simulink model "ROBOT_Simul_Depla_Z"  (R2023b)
settings: Solver=ode15s  StartTime=0.0  StopTime=0.2  RelTol=1e-3  EnableMultiTasking=on
undefined symbols (not defined in the file): BATI1_Défaut_sldprt, BATI2_Défaut_sldprt, BATI3_Défaut_sldprt, deg, kg, m, mm, N, rad, s, STL, X, Y, Z
libraries: sm_lib x139, fl_lib x42, nesl_utility x19, slpidlib x3
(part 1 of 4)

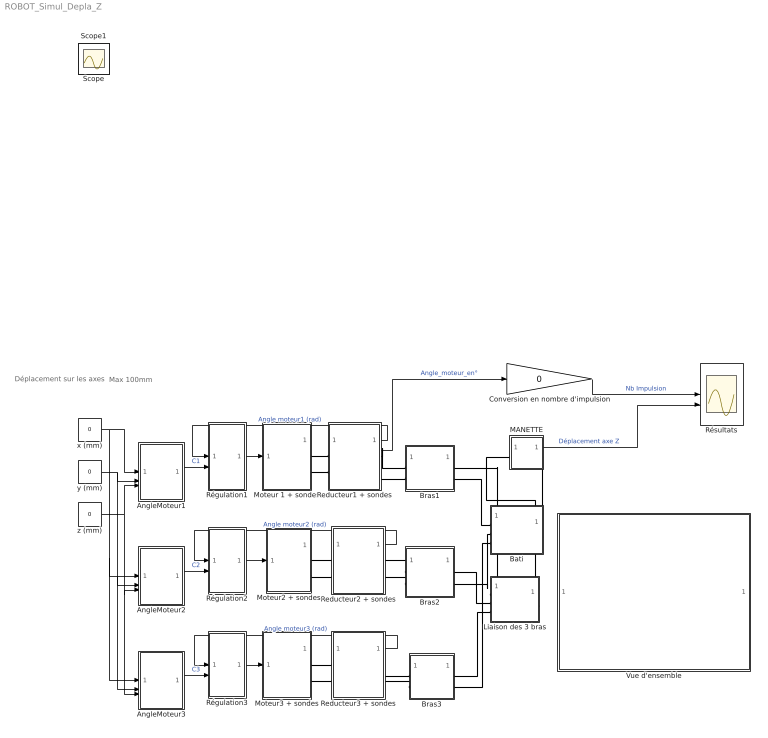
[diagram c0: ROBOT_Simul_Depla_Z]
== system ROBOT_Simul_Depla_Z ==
  note: Déplacement sur les axes
  note: Max 100mm
  AngleMoteur1 : MATLAB Function  TreatAsAtomicUnit=on
  AngleMoteur2 : MATLAB Function  TreatAsAtomicUnit=on
  AngleMoteur3 : MATLAB Function  TreatAsAtomicUnit=on
  Bati : Subsystem
  Bras1 : Subsystem
  Bras2 : Subsystem
  Bras3 : Subsystem
  Conversion en nombre d'impulsion : Gain  Gain=0
  Liaison des 3 bras : Subsystem
  MANETTE : Subsystem
  Moteur 1 + sondes : Subsystem
  Moteur2 + sondes : Subsystem
  Moteur3 + sondes : Subsystem
  Reducteur1 + sondes : Subsystem
  Reducteur2 + sondes : Subsystem
  Reducteur3 + sondes : Subsystem
  Régulation1 : Subsystem
  Régulation2 : Subsystem
  Régulation3 : Subsystem
  Résultats : Scope  NumInputPorts=2
  Vue d'ensemble : Subsystem
  x (mm) : Constant  Value=0
  y (mm) : Constant  Value=0
  z (mm) : Constant  Value=0
  Scope : Scope
  Scope1 : Scope
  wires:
  Régulation3/1(Out1) -> Moteur3 + sondes/1(In1)
  Reducteur3 + sondes/1(Angle_mot3) -> Régulation3/1(In1)  "Angle moteur3 (rad)"
  Régulation1/1(Out1) -> Moteur 1 + sondes/1(In1)
  Reducteur1 + sondes/1(Angle_mot1) -> Régulation1/1(In1)  "Angle moteur1 (rad)"
  Régulation2/1(Out1) -> Moteur2 + sondes/1(In1)
  Reducteur2 + sondes/1(Angle_mot2) -> Régulation2/1(In1)  "Angle moteur2 (rad)"
  AngleMoteur3/1(anglmot3) -> Régulation3/2(In2)  "C3"
  x (mm)/1 -> AngleMoteur1/1(x), AngleMoteur2/1(x), AngleMoteur3/1(x)
  AngleMoteur1/1(anglmot1) -> Régulation1/2(In2)  "C1"
  AngleMoteur2/1(anglmot2) -> Régulation2/2(In2)  "C2"
  y (mm)/1 -> AngleMoteur1/2(y), AngleMoteur2/2(y), AngleMoteur3/2(y)
  z (mm)/1 -> AngleMoteur1/3(z), AngleMoteur2/3(z), AngleMoteur3/3(z)
  Reducteur1 + sondes/2(Angle_mot_°) -> Conversion en nombre d'impulsion/1  "Angle_moteur_en°"
  Conversion en nombre d'impulsion/1 -> Résultats/1  "Nb Impulsion"
  MANETTE/1(Out1) -> Résultats/2  "Déplacement axe Z"
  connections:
  Liaison des 3 bras/RConn1 -- MANETTE/LConn1
  Moteur3 + sondes/RConn1 -- Reducteur3 + sondes/LConn1
  Moteur 1 + sondes/RConn1 -- Reducteur1 + sondes/LConn1
  Moteur3 + sondes/RConn2 -- Reducteur3 + sondes/LConn2
  Reducteur1 + sondes/LConn2 -- Moteur 1 + sondes/RConn2
  Moteur2 + sondes/RConn2 -- Reducteur2 + sondes/LConn2
  Moteur2 + sondes/RConn1 -- Reducteur2 + sondes/LConn1
  Reducteur1 + sondes/RConn1 -- Bras1/LConn1
  Reducteur1 + sondes/RConn2 -- Bras1/LConn2
  Liaison des 3 bras/LConn1 -- Bras1/RConn1
  Liaison des 3 bras/LConn2 -- Bras2/RConn1
  Bras2/LConn1 -- Reducteur2 + sondes/RConn1
  Bras2/LConn2 -- Reducteur2 + sondes/RConn2
  Liaison des 3 bras/LConn3 -- Bras3/RConn1
  Reducteur3 + sondes/RConn1 -- Bras3/LConn1
  Bras3/LConn2 -- Reducteur3 + sondes/RConn2
  Bati/LConn1 -- Bras1/RConn2
  Bati/LConn2 -- Bras2/RConn2
  Bati/LConn3 -- Bras3/RConn2
  MANETTE/RConn1 -- Bati/RConn1

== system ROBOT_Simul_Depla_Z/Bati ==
  BATI_1_RIGID : Subsystem
  MechanismConfiguration : sm_lib/Utilities/Mechanism Configuration  UniformGravity=Constant  GravityVector=[0 -9.81 0]  GravityVectorUnits=m/s^2  LinearizationDelta=0.001  JointModeTransitionNonlinearIterations=2
  Solver Configuration : nesl_utility/Solver Configuration  PhysicalDomain=network_engine_domain  SubClassName=solver  LeftPortType=input  RightPortType=generic  Tones=[]  Harmonics=[]  SimulateNoise=off  Profile=off  UseLocalSampling=off  EnableSwitchedLinearOptims=on  FrequencyDomain=off  UseCCode=off  RelTol=0.001  AbsTol=1e-06  MinStep=1e-09  ToWorkspace=off  RevertToSquareIcSolve=off  NumHomotopyIterations=100  PhasorMode=off  PhasorModeNumHarmonics=1  ConsistencySolver=NEWTON_FTOL  IndexReductionMethod=DerivativeReplacement  DoDC=off  ResidualTolerance=1e-09  ConsistencyTolSource=GLOBAL  ConsistencyAbsTol=0.001  ConsistencyRelTol=0.001  ConsistencyTolFactor=0.001  UseLocalSolver=off  LocalSolverChoice=NE_BACKWARD_EULER_ADVANCER  ResolveIndetEquations=on  FunctionEvalNumThread=1  LocalSolverSampleTime=0.001  DoFixedCost=off  MaxNonlinIter=3  MaxModeIter=2  ComputeImpulses=off  ImpulseIterations=2  LinearAlgebra=Sparse  LinearAlgebraNumThread=0  EquationFormulation=NE_TIME_EF  DelaysMemoryBudget=1024  AutomaticFiltering=on  FilteringTimeConstant=0.001  PartitionStorageMethod=AS_NEEDED  PartitionMemoryBudget=1024  PartitionMethod=FAST  MultibodyUseLocalSolver=off  MultibodyLocalSolverChoice=ODE1  MultibodyLocalSolverSampleTime=0.001
  Transform : sm_lib/Frames and Transforms/Rigid Transform  TranslationMethod=Cartesian  TranslationStandardOffset=0  TranslationStandardOffsetUnits=mm  TranslationStandardAxis=+Z  TranslationCartesianOffset=[14.920329062241711 -30.551170260312524 -19.999999999988649]  TranslationCartesianOffsetUnits=mm  TranslationROffset=0  TranslationROffsetUnits=m  TranslationZOffset=0  TranslationZOffsetUnits=m  TranslationThetaOffset=0  TranslationThetaOffsetUnits=deg  RotationMethod=ArbitraryAxis  RotationAngleUnits=rad  RotationStandardAxis=+Z  RotationAngle=1.8228218707828856  RotationArbitraryAxis=[4.4011854841110467e-16 1.1162668393823967e-16 -1]  FollAlignAxisA=+X  BaseAlignAxisA=+Y  FollAlignAxisB=+Y  BaseAlignAxisB=+Z  RotationSequenceAxes=FollowerAxes  RotationSequence=XYX  RotationSequenceAngles=[0 0 0]  RotationSequenceAnglesUnits=deg  RotationMatrix=[1 0 0; 0 1 0; 0 0 1]  Quaternion=[1 0 0 0]
  World : sm_lib/Frames and Transforms/World Frame
  E1 : PMIOPort  Side=Left
  E2 : PMIOPort  Port=2  Side=Left
  E3 : PMIOPort  Port=3  Side=Left
  Wrld : PMIOPort  Port=4  Side=Right
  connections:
  Transform/LConn1 -- MechanismConfiguration/RConn1 -- Wrld/RConn1 -- World/RConn1 -- Solver Configuration/RConn1
  BATI_1_RIGID/LConn1 -- Transform/RConn1
  BATI_1_RIGID/RConn3 -- E1/RConn1
  BATI_1_RIGID/RConn1 -- E3/RConn1
  BATI_1_RIGID/RConn2 -- E2/RConn1

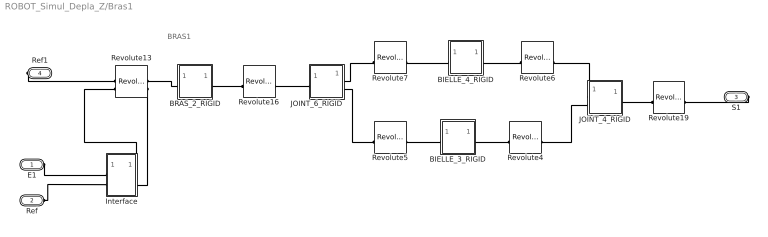
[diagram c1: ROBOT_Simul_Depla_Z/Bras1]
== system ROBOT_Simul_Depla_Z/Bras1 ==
  note: BRAS1
  BIELLE_3_RIGID : Subsystem
  BIELLE_4_RIGID : Subsystem
  BRAS_2_RIGID : Subsystem
  Interface : Subsystem
  JOINT_4_RIGID : Subsystem
  JOINT_6_RIGID : Subsystem
  Revolute13 : sm_lib/Joints/Revolute Joint  JointMode=Normal  SenseConstraintForce=off  SenseConstraintForceX=off  SenseConstraintForceY=off  SenseConstraintForceZ=off  SenseConstraintTorque=off  SenseConstraintTorqueX=off  SenseConstraintTorqueY=off  SenseConstraintTorqueZ=off  SenseTotalForce=off  SenseTotalForceX=off  SenseTotalForceY=off  SenseTotalForceZ=off  SenseTotalTorque=off  SenseTotalTorqueX=off  SenseTotalTorqueY=off  SenseTotalTorqueZ=off  CompositeWrenchDir=FollowerOnBase  CompositeWrenchFrame=BaseFrame  EquilibriumPosition=0  EquilibriumPositionUnits=rad  SpringStiffness=0  SpringStiffnessUnits=m*N/rad  DampingCoefficient=0  DampingCoefficientUnits=m*s*N/rad  TorqueActuationMode=InputTorque  MotionActuationMode=ComputedMotion  SensePosition=off  SenseVelocity=on  SenseAcceleration=off  SenseTorqueForce=off  SenseLowerLimitTorqueForce=off  SenseUpperLimitTorqueForce=off  LowerLimitSpecify=off  LowerLimitBound=-90  LowerLimitBoundUnits=deg  LowerLimitStiffness=1e4  LowerLimitStiffnessUnits=N*m/deg  LowerLimitDamping=10  LowerLimitDampingUnits=N*m/(deg/s)  LowerLimitTransitionRegionWidth=0.1  LowerLimitTransitionRegionWidthUnits=deg  UpperLimitSpecify=off  UpperLimitBound=90  UpperLimitBoundUnits=deg  UpperLimitStiffness=1e4  UpperLimitStiffnessUnits=N*m/deg  UpperLimitDamping=10  UpperLimitDampingUnits=N*m/(deg/s)  UpperLimitTransitionRegionWidth=0.1  UpperLimitTransitionRegionWidthUnits=deg  PositionTargetSpecify=on  PositionTargetPriority=Low  PositionTargetValue=11.887378711744704  PositionTargetValueUnits=deg  VelocityTargetSpecify=off  VelocityTargetPriority=High  VelocityTargetValue=0  VelocityTargetValueUnits=deg/s
  Revolute16 : sm_lib/Joints/Revolute Joint  JointMode=Normal  SenseConstraintForce=off  SenseConstraintForceX=off  SenseConstraintForceY=off  SenseConstraintForceZ=off  SenseConstraintTorque=off  SenseConstraintTorqueX=off  SenseConstraintTorqueY=off  SenseConstraintTorqueZ=off  SenseTotalForce=off  SenseTotalForceX=off  SenseTotalForceY=off  SenseTotalForceZ=off  SenseTotalTorque=off  SenseTotalTorqueX=off  SenseTotalTorqueY=off  SenseTotalTorqueZ=off  CompositeWrenchDir=FollowerOnBase  CompositeWrenchFrame=BaseFrame  EquilibriumPosition=0  EquilibriumPositionUnits=rad  SpringStiffness=0  SpringStiffnessUnits=m*N/rad  DampingCoefficient=0  DampingCoefficientUnits=m*s*N/rad  TorqueActuationMode=NoTorque  MotionActuationMode=ComputedMotion  SensePosition=off  SenseVelocity=off  SenseAcceleration=off  SenseTorqueForce=off  SenseLowerLimitTorqueForce=off  SenseUpperLimitTorqueForce=off  LowerLimitSpecify=off  LowerLimitBound=-90  LowerLimitBoundUnits=deg  LowerLimitStiffness=1e4  LowerLimitStiffnessUnits=N*m/deg  LowerLimitDamping=10  LowerLimitDampingUnits=N*m/(deg/s)  LowerLimitTransitionRegionWidth=0.1  LowerLimitTransitionRegionWidthUnits=deg  UpperLimitSpecify=off  UpperLimitBound=90  UpperLimitBoundUnits=deg  UpperLimitStiffness=1e4  UpperLimitStiffnessUnits=N*m/deg  UpperLimitDamping=10  UpperLimitDampingUnits=N*m/(deg/s)  UpperLimitTransitionRegionWidth=0.1  UpperLimitTransitionRegionWidthUnits=deg  PositionTargetSpecify=on  PositionTargetPriority=Low  PositionTargetValue=-127.14100786995047  PositionTargetValueUnits=deg  VelocityTargetSpecify=off  VelocityTargetPriority=High  VelocityTargetValue=0  VelocityTargetValueUnits=deg/s
  Revolute19 : sm_lib/Joints/Revolute Joint  JointMode=Normal  SenseConstraintForce=off  SenseConstraintForceX=off  SenseConstraintForceY=off  SenseConstraintForceZ=off  SenseConstraintTorque=off  SenseConstraintTorqueX=off  SenseConstraintTorqueY=off  SenseConstraintTorqueZ=off  SenseTotalForce=off  SenseTotalForceX=off  SenseTotalForceY=off  SenseTotalForceZ=off  SenseTotalTorque=off  SenseTotalTorqueX=off  SenseTotalTorqueY=off  SenseTotalTorqueZ=off  CompositeWrenchDir=FollowerOnBase  CompositeWrenchFrame=BaseFrame  EquilibriumPosition=0  EquilibriumPositionUnits=rad  SpringStiffness=0  SpringStiffnessUnits=m*N/rad  DampingCoefficient=0  DampingCoefficientUnits=m*s*N/rad  TorqueActuationMode=NoTorque  MotionActuationMode=ComputedMotion  SensePosition=off  SenseVelocity=off  SenseAcceleration=off  SenseTorqueForce=off  SenseLowerLimitTorqueForce=off  SenseUpperLimitTorqueForce=off  LowerLimitSpecify=off  LowerLimitBound=-90  LowerLimitBoundUnits=deg  LowerLimitStiffness=1e4  LowerLimitStiffnessUnits=N*m/deg  LowerLimitDamping=10  LowerLimitDampingUnits=N*m/(deg/s)  LowerLimitTransitionRegionWidth=0.1  LowerLimitTransitionRegionWidthUnits=deg  UpperLimitSpecify=off  UpperLimitBound=90  UpperLimitBoundUnits=deg  UpperLimitStiffness=1e4  UpperLimitStiffnessUnits=N*m/deg  UpperLimitDamping=10  UpperLimitDampingUnits=N*m/(deg/s)  UpperLimitTransitionRegionWidth=0.1  UpperLimitTransitionRegionWidthUnits=deg  PositionTargetSpecify=off  PositionTargetPriority=High  PositionTargetValue=0  PositionTargetValueUnits=deg  VelocityTargetSpecify=off  VelocityTargetPriority=High  VelocityTargetValue=0  VelocityTargetValueUnits=deg/s
  Revolute4 : sm_lib/Joints/Revolute Joint  JointMode=Normal  SenseConstraintForce=off  SenseConstraintForceX=off  SenseConstraintForceY=off  SenseConstraintForceZ=off  SenseConstraintTorque=off  SenseConstraintTorqueX=off  SenseConstraintTorqueY=off  SenseConstraintTorqueZ=off  SenseTotalForce=off  SenseTotalForceX=off  SenseTotalForceY=off  SenseTotalForceZ=off  SenseTotalTorque=off  SenseTotalTorqueX=off  SenseTotalTorqueY=off  SenseTotalTorqueZ=off  CompositeWrenchDir=FollowerOnBase  CompositeWrenchFrame=BaseFrame  EquilibriumPosition=0  EquilibriumPositionUnits=rad  SpringStiffness=0  SpringStiffnessUnits=m*N/rad  DampingCoefficient=0  DampingCoefficientUnits=m*s*N/rad  TorqueActuationMode=NoTorque  MotionActuationMode=ComputedMotion  SensePosition=off  SenseVelocity=off  SenseAcceleration=off  SenseTorqueForce=off  SenseLowerLimitTorqueForce=off  SenseUpperLimitTorqueForce=off  LowerLimitSpecify=off  LowerLimitBound=-90  LowerLimitBoundUnits=deg  LowerLimitStiffness=1e4  LowerLimitStiffnessUnits=N*m/deg  LowerLimitDamping=10  LowerLimitDampingUnits=N*m/(deg/s)  LowerLimitTransitionRegionWidth=0.1  LowerLimitTransitionRegionWidthUnits=deg  UpperLimitSpecify=off  UpperLimitBound=90  UpperLimitBoundUnits=deg  UpperLimitStiffness=1e4  UpperLimitStiffnessUnits=N*m/deg  UpperLimitDamping=10  UpperLimitDampingUnits=N*m/(deg/s)  UpperLimitTransitionRegionWidth=0.1  UpperLimitTransitionRegionWidthUnits=deg  PositionTargetSpecify=on  PositionTargetPriority=Low  PositionTargetValue=-91.30254308411611  PositionTargetValueUnits=deg  VelocityTargetSpecify=off  VelocityTargetPriority=High  VelocityTargetValue=0  VelocityTargetValueUnits=deg/s
  Revolute5 : sm_lib/Joints/Revolute Joint  JointMode=Normal  SenseConstraintForce=off  SenseConstraintForceX=off  SenseConstraintForceY=off  SenseConstraintForceZ=off  SenseConstraintTorque=off  SenseConstraintTorqueX=off  SenseConstraintTorqueY=off  SenseConstraintTorqueZ=off  SenseTotalForce=off  SenseTotalForceX=off  SenseTotalForceY=off  SenseTotalForceZ=off  SenseTotalTorque=off  SenseTotalTorqueX=off  SenseTotalTorqueY=off  SenseTotalTorqueZ=off  CompositeWrenchDir=FollowerOnBase  CompositeWrenchFrame=BaseFrame  EquilibriumPosition=0  EquilibriumPositionUnits=rad  SpringStiffness=0  SpringStiffnessUnits=m*N/rad  DampingCoefficient=0  DampingCoefficientUnits=m*s*N/rad  TorqueActuationMode=NoTorque  MotionActuationMode=ComputedMotion  SensePosition=off  SenseVelocity=off  SenseAcceleration=off  SenseTorqueForce=off  SenseLowerLimitTorqueForce=off  SenseUpperLimitTorqueForce=off  LowerLimitSpecify=off  LowerLimitBound=-90  LowerLimitBoundUnits=deg  LowerLimitStiffness=1e4  LowerLimitStiffnessUnits=N*m/deg  LowerLimitDamping=10  LowerLimitDampingUnits=N*m/(deg/s)  LowerLimitTransitionRegionWidth=0.1  LowerLimitTransitionRegionWidthUnits=deg  UpperLimitSpecify=off  UpperLimitBound=90  UpperLimitBoundUnits=deg  UpperLimitStiffness=1e4  UpperLimitStiffnessUnits=N*m/deg  UpperLimitDamping=10  UpperLimitDampingUnits=N*m/(deg/s)  UpperLimitTransitionRegionWidth=0.1  UpperLimitTransitionRegionWidthUnits=deg  PositionTargetSpecify=on  PositionTargetPriority=Low  PositionTargetValue=-91.302543084116394  PositionTargetValueUnits=deg  VelocityTargetSpecify=off  VelocityTargetPriority=High  VelocityTargetValue=0  VelocityTargetValueUnits=deg/s
  Revolute6 : sm_lib/Joints/Revolute Joint  JointMode=Normal  SenseConstraintForce=off  SenseConstraintForceX=off  SenseConstraintForceY=off  SenseConstraintForceZ=off  SenseConstraintTorque=off  SenseConstraintTorqueX=off  SenseConstraintTorqueY=off  SenseConstraintTorqueZ=off  SenseTotalForce=off  SenseTotalForceX=off  SenseTotalForceY=off  SenseTotalForceZ=off  SenseTotalTorque=off  SenseTotalTorqueX=off  SenseTotalTorqueY=off  SenseTotalTorqueZ=off  CompositeWrenchDir=FollowerOnBase  CompositeWrenchFrame=BaseFrame  EquilibriumPosition=0  EquilibriumPositionUnits=rad  SpringStiffness=0  SpringStiffnessUnits=m*N/rad  DampingCoefficient=0  DampingCoefficientUnits=m*s*N/rad  TorqueActuationMode=NoTorque  MotionActuationMode=ComputedMotion  SensePosition=off  SenseVelocity=off  SenseAcceleration=off  SenseTorqueForce=off  SenseLowerLimitTorqueForce=off  SenseUpperLimitTorqueForce=off  LowerLimitSpecify=off  LowerLimitBound=-90  LowerLimitBoundUnits=deg  LowerLimitStiffness=1e4  LowerLimitStiffnessUnits=N*m/deg  LowerLimitDamping=10  LowerLimitDampingUnits=N*m/(deg/s)  LowerLimitTransitionRegionWidth=0.1  LowerLimitTransitionRegionWidthUnits=deg  UpperLimitSpecify=off  UpperLimitBound=90  UpperLimitBoundUnits=deg  UpperLimitStiffness=1e4  UpperLimitStiffnessUnits=N*m/deg  UpperLimitDamping=10  UpperLimitDampingUnits=N*m/(deg/s)  UpperLimitTransitionRegionWidth=0.1  UpperLimitTransitionRegionWidthUnits=deg  PositionTargetSpecify=off  PositionTargetPriority=High  PositionTargetValue=0  PositionTargetValueUnits=deg  VelocityTargetSpecify=off  VelocityTargetPriority=High  VelocityTargetValue=0  VelocityTargetValueUnits=deg/s
  Revolute7 : sm_lib/Joints/Revolute Joint  JointMode=Normal  SenseConstraintForce=off  SenseConstraintForceX=off  SenseConstraintForceY=off  SenseConstraintForceZ=off  SenseConstraintTorque=off  SenseConstraintTorqueX=off  SenseConstraintTorqueY=off  SenseConstraintTorqueZ=off  SenseTotalForce=off  SenseTotalForceX=off  SenseTotalForceY=off  SenseTotalForceZ=off  SenseTotalTorque=off  SenseTotalTorqueX=off  SenseTotalTorqueY=off  SenseTotalTorqueZ=off  CompositeWrenchDir=FollowerOnBase  CompositeWrenchFrame=BaseFrame  EquilibriumPosition=0  EquilibriumPositionUnits=rad  SpringStiffness=0  SpringStiffnessUnits=m*N/rad  DampingCoefficient=0  DampingCoefficientUnits=m*s*N/rad  TorqueActuationMode=NoTorque  MotionActuationMode=ComputedMotion  SensePosition=off  SenseVelocity=off  SenseAcceleration=off  SenseTorqueForce=off  SenseLowerLimitTorqueForce=off  SenseUpperLimitTorqueForce=off  LowerLimitSpecify=off  LowerLimitBound=-90  LowerLimitBoundUnits=deg  LowerLimitStiffness=1e4  LowerLimitStiffnessUnits=N*m/deg  LowerLimitDamping=10  LowerLimitDampingUnits=N*m/(deg/s)  LowerLimitTransitionRegionWidth=0.1  LowerLimitTransitionRegionWidthUnits=deg  UpperLimitSpecify=off  UpperLimitBound=90  UpperLimitBoundUnits=deg  UpperLimitStiffness=1e4  UpperLimitStiffnessUnits=N*m/deg  UpperLimitDamping=10  UpperLimitDampingUnits=N*m/(deg/s)  UpperLimitTransitionRegionWidth=0.1  UpperLimitTransitionRegionWidthUnits=deg  PositionTargetSpecify=on  PositionTargetPriority=Low  PositionTargetValue=91.302543084116408  PositionTargetValueUnits=deg  VelocityTargetSpecify=off  VelocityTargetPriority=High  VelocityTargetValue=0  VelocityTargetValueUnits=deg/s
  E1 : PMIOPort  Side=Left
  Ref : PMIOPort  Port=2  Side=Left
  S1 : PMIOPort  Port=3  Side=Right
  Ref1 : PMIOPort  Port=4  Side=Right
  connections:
  JOINT_4_RIGID/LConn2 -- Revolute4/RConn1
  BIELLE_4_RIGID/LConn1 -- Revolute7/LConn1
  BIELLE_3_RIGID/LConn1 -- Revolute5/LConn1
  JOINT_6_RIGID/RConn2 -- Revolute5/RConn1
  BIELLE_4_RIGID/RConn1 -- Revolute6/LConn1
  JOINT_4_RIGID/LConn1 -- Revolute6/RConn1
  BRAS_2_RIGID/RConn1 -- Revolute16/LConn1
  S1/RConn1 -- Revolute19/LConn1
  BRAS_2_RIGID/LConn1 -- Revolute13/RConn1
  JOINT_4_RIGID/RConn1 -- Revolute19/RConn1
  JOINT_6_RIGID/LConn1 -- Revolute16/RConn1
  Ref1/RConn1 -- Revolute13/LConn1
  JOINT_6_RIGID/RConn1 -- Revolute7/RConn1
  BIELLE_3_RIGID/RConn1 -- Revolute4/LConn1
  Interface/RConn1 -- Revolute13/LConn2
  Interface/RConn2 -- Revolute13/RConn2
  E1/RConn1 -- Interface/LConn1
  Ref/RConn1 -- Interface/LConn2

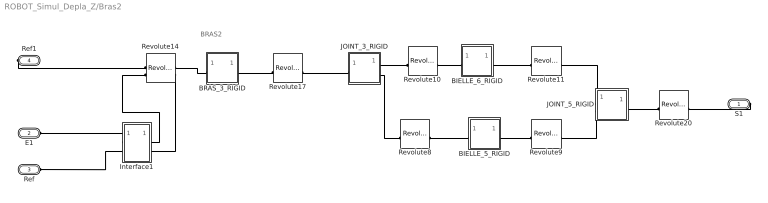
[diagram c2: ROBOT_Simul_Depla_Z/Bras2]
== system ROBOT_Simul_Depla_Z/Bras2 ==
  note: BRAS2
  BIELLE_5_RIGID : Subsystem
  BIELLE_6_RIGID : Subsystem
  BRAS_3_RIGID : Subsystem
  Interface1 : Subsystem
  JOINT_3_RIGID : Subsystem
  JOINT_5_RIGID : Subsystem
  Revolute10 : sm_lib/Joints/Revolute Joint  JointMode=Normal  SenseConstraintForce=off  SenseConstraintForceX=off  SenseConstraintForceY=off  SenseConstraintForceZ=off  SenseConstraintTorque=off  SenseConstraintTorqueX=off  SenseConstraintTorqueY=off  SenseConstraintTorqueZ=off  SenseTotalForce=off  SenseTotalForceX=off  SenseTotalForceY=off  SenseTotalForceZ=off  SenseTotalTorque=off  SenseTotalTorqueX=off  SenseTotalTorqueY=off  SenseTotalTorqueZ=off  CompositeWrenchDir=FollowerOnBase  CompositeWrenchFrame=BaseFrame  EquilibriumPosition=0  EquilibriumPositionUnits=rad  SpringStiffness=0  SpringStiffnessUnits=m*N/rad  DampingCoefficient=0  DampingCoefficientUnits=m*s*N/rad  TorqueActuationMode=NoTorque  MotionActuationMode=ComputedMotion  SensePosition=off  SenseVelocity=off  SenseAcceleration=off  SenseTorqueForce=off  SenseLowerLimitTorqueForce=off  SenseUpperLimitTorqueForce=off  LowerLimitSpecify=off  LowerLimitBound=-90  LowerLimitBoundUnits=deg  LowerLimitStiffness=1e4  LowerLimitStiffnessUnits=N*m/deg  LowerLimitDamping=10  LowerLimitDampingUnits=N*m/(deg/s)  LowerLimitTransitionRegionWidth=0.1  LowerLimitTransitionRegionWidthUnits=deg  UpperLimitSpecify=off  UpperLimitBound=90  UpperLimitBoundUnits=deg  UpperLimitStiffness=1e4  UpperLimitStiffnessUnits=N*m/deg  UpperLimitDamping=10  UpperLimitDampingUnits=N*m/(deg/s)  UpperLimitTransitionRegionWidth=0.1  UpperLimitTransitionRegionWidthUnits=deg  PositionTargetSpecify=on  PositionTargetPriority=Low  PositionTargetValue=-88.697456915883507  PositionTargetValueUnits=deg  VelocityTargetSpecify=off  VelocityTargetPriority=High  VelocityTargetValue=0  VelocityTargetValueUnits=deg/s
  Revolute11 : sm_lib/Joints/Revolute Joint  JointMode=Normal  SenseConstraintForce=off  SenseConstraintForceX=off  SenseConstraintForceY=off  SenseConstraintForceZ=off  SenseConstraintTorque=off  SenseConstraintTorqueX=off  SenseConstraintTorqueY=off  SenseConstraintTorqueZ=off  SenseTotalForce=off  SenseTotalForceX=off  SenseTotalForceY=off  SenseTotalForceZ=off  SenseTotalTorque=off  SenseTotalTorqueX=off  SenseTotalTorqueY=off  SenseTotalTorqueZ=off  CompositeWrenchDir=FollowerOnBase  CompositeWrenchFrame=BaseFrame  EquilibriumPosition=0  EquilibriumPositionUnits=rad  SpringStiffness=0  SpringStiffnessUnits=m*N/rad  DampingCoefficient=0  DampingCoefficientUnits=m*s*N/rad  TorqueActuationMode=NoTorque  MotionActuationMode=ComputedMotion  SensePosition=off  SenseVelocity=off  SenseAcceleration=off  SenseTorqueForce=off  SenseLowerLimitTorqueForce=off  SenseUpperLimitTorqueForce=off  LowerLimitSpecify=off  LowerLimitBound=-90  LowerLimitBoundUnits=deg  LowerLimitStiffness=1e4  LowerLimitStiffnessUnits=N*m/deg  LowerLimitDamping=10  LowerLimitDampingUnits=N*m/(deg/s)  LowerLimitTransitionRegionWidth=0.1  LowerLimitTransitionRegionWidthUnits=deg  UpperLimitSpecify=off  UpperLimitBound=90  UpperLimitBoundUnits=deg  UpperLimitStiffness=1e4  UpperLimitStiffnessUnits=N*m/deg  UpperLimitDamping=10  UpperLimitDampingUnits=N*m/(deg/s)  UpperLimitTransitionRegionWidth=0.1  UpperLimitTransitionRegionWidthUnits=deg  PositionTargetSpecify=off  PositionTargetPriority=High  PositionTargetValue=0  PositionTargetValueUnits=deg  VelocityTargetSpecify=off  VelocityTargetPriority=High  VelocityTargetValue=0  VelocityTargetValueUnits=deg/s
  Revolute14 : sm_lib/Joints/Revolute Joint  JointMode=Normal  SenseConstraintForce=off  SenseConstraintForceX=off  SenseConstraintForceY=off  SenseConstraintForceZ=off  SenseConstraintTorque=off  SenseConstraintTorqueX=off  SenseConstraintTorqueY=off  SenseConstraintTorqueZ=off  SenseTotalForce=off  SenseTotalForceX=off  SenseTotalForceY=off  SenseTotalForceZ=off  SenseTotalTorque=off  SenseTotalTorqueX=off  SenseTotalTorqueY=off  SenseTotalTorqueZ=off  CompositeWrenchDir=FollowerOnBase  CompositeWrenchFrame=BaseFrame  EquilibriumPosition=0  EquilibriumPositionUnits=rad  SpringStiffness=0  SpringStiffnessUnits=m*N/rad  DampingCoefficient=0  DampingCoefficientUnits=m*s*N/rad  TorqueActuationMode=InputTorque  MotionActuationMode=ComputedMotion  SensePosition=off  SenseVelocity=on  SenseAcceleration=off  SenseTorqueForce=off  SenseLowerLimitTorqueForce=off  SenseUpperLimitTorqueForce=off  LowerLimitSpecify=off  LowerLimitBound=-90  LowerLimitBoundUnits=deg  LowerLimitStiffness=1e4  LowerLimitStiffnessUnits=N*m/deg  LowerLimitDamping=10  LowerLimitDampingUnits=N*m/(deg/s)  LowerLimitTransitionRegionWidth=0.1  LowerLimitTransitionRegionWidthUnits=deg  UpperLimitSpecify=off  UpperLimitBound=90  UpperLimitBoundUnits=deg  UpperLimitStiffness=1e4  UpperLimitStiffnessUnits=N*m/deg  UpperLimitDamping=10  UpperLimitDampingUnits=N*m/(deg/s)  UpperLimitTransitionRegionWidth=0.1  UpperLimitTransitionRegionWidthUnits=deg  PositionTargetSpecify=on  PositionTargetPriority=Low  PositionTargetValue=-168.11262128825132  PositionTargetValueUnits=deg  VelocityTargetSpecify=off  VelocityTargetPriority=High  VelocityTargetValue=0  VelocityTargetValueUnits=deg/s
  Revolute17 : sm_lib/Joints/Revolute Joint  JointMode=Normal  SenseConstraintForce=off  SenseConstraintForceX=off  SenseConstraintForceY=off  SenseConstraintForceZ=off  SenseConstraintTorque=off  SenseConstraintTorqueX=off  SenseConstraintTorqueY=off  SenseConstraintTorqueZ=off  SenseTotalForce=off  SenseTotalForceX=off  SenseTotalForceY=off  SenseTotalForceZ=off  SenseTotalTorque=off  SenseTotalTorqueX=off  SenseTotalTorqueY=off  SenseTotalTorqueZ=off  CompositeWrenchDir=FollowerOnBase  CompositeWrenchFrame=BaseFrame  EquilibriumPosition=0  EquilibriumPositionUnits=rad  SpringStiffness=0  SpringStiffnessUnits=m*N/rad  DampingCoefficient=0  DampingCoefficientUnits=m*s*N/rad  TorqueActuationMode=NoTorque  MotionActuationMode=ComputedMotion  SensePosition=off  SenseVelocity=off  SenseAcceleration=off  SenseTorqueForce=off  SenseLowerLimitTorqueForce=off  SenseUpperLimitTorqueForce=off  LowerLimitSpecify=off  LowerLimitBound=-90  LowerLimitBoundUnits=deg  LowerLimitStiffness=1e4  LowerLimitStiffnessUnits=N*m/deg  LowerLimitDamping=10  LowerLimitDampingUnits=N*m/(deg/s)  LowerLimitTransitionRegionWidth=0.1  LowerLimitTransitionRegionWidthUnits=deg  UpperLimitSpecify=off  UpperLimitBound=90  UpperLimitBoundUnits=deg  UpperLimitStiffness=1e4  UpperLimitStiffnessUnits=N*m/deg  UpperLimitDamping=10  UpperLimitDampingUnits=N*m/(deg/s)  UpperLimitTransitionRegionWidth=0.1  UpperLimitTransitionRegionWidthUnits=deg  PositionTargetSpecify=on  PositionTargetPriority=Low  PositionTargetValue=-52.858992130053309  PositionTargetValueUnits=deg  VelocityTargetSpecify=off  VelocityTargetPriority=High  VelocityTargetValue=0  VelocityTargetValueUnits=deg/s
  Revolute20 : sm_lib/Joints/Revolute Joint  JointMode=Normal  SenseConstraintForce=off  SenseConstraintForceX=off  SenseConstraintForceY=off  SenseConstraintForceZ=off  SenseConstraintTorque=off  SenseConstraintTorqueX=off  SenseConstraintTorqueY=off  SenseConstraintTorqueZ=off  SenseTotalForce=off  SenseTotalForceX=off  SenseTotalForceY=off  SenseTotalForceZ=off  SenseTotalTorque=off  SenseTotalTorqueX=off  SenseTotalTorqueY=off  SenseTotalTorqueZ=off  CompositeWrenchDir=FollowerOnBase  CompositeWrenchFrame=BaseFrame  EquilibriumPosition=0  EquilibriumPositionUnits=rad  SpringStiffness=0  SpringStiffnessUnits=m*N/rad  DampingCoefficient=0  DampingCoefficientUnits=m*s*N/rad  TorqueActuationMode=NoTorque  MotionActuationMode=ComputedMotion  SensePosition=off  SenseVelocity=off  SenseAcceleration=off  SenseTorqueForce=off  SenseLowerLimitTorqueForce=off  SenseUpperLimitTorqueForce=off  LowerLimitSpecify=off  LowerLimitBound=-90  LowerLimitBoundUnits=deg  LowerLimitStiffness=1e4  LowerLimitStiffnessUnits=N*m/deg  LowerLimitDamping=10  LowerLimitDampingUnits=N*m/(deg/s)  LowerLimitTransitionRegionWidth=0.1  LowerLimitTransitionRegionWidthUnits=deg  UpperLimitSpecify=off  UpperLimitBound=90  UpperLimitBoundUnits=deg  UpperLimitStiffness=1e4  UpperLimitStiffnessUnits=N*m/deg  UpperLimitDamping=10  UpperLimitDampingUnits=N*m/(deg/s)  UpperLimitTransitionRegionWidth=0.1  UpperLimitTransitionRegionWidthUnits=deg  PositionTargetSpecify=off  PositionTargetPriority=High  PositionTargetValue=0  PositionTargetValueUnits=deg  VelocityTargetSpecify=off  VelocityTargetPriority=High  VelocityTargetValue=0  VelocityTargetValueUnits=deg/s
  Revolute8 : sm_lib/Joints/Revolute Joint  JointMode=Normal  SenseConstraintForce=off  SenseConstraintForceX=off  SenseConstraintForceY=off  SenseConstraintForceZ=off  SenseConstraintTorque=off  SenseConstraintTorqueX=off  SenseConstraintTorqueY=off  SenseConstraintTorqueZ=off  SenseTotalForce=off  SenseTotalForceX=off  SenseTotalForceY=off  SenseTotalForceZ=off  SenseTotalTorque=off  SenseTotalTorqueX=off  SenseTotalTorqueY=off  SenseTotalTorqueZ=off  CompositeWrenchDir=FollowerOnBase  CompositeWrenchFrame=BaseFrame  EquilibriumPosition=0  EquilibriumPositionUnits=rad  SpringStiffness=0  SpringStiffnessUnits=m*N/rad  DampingCoefficient=0  DampingCoefficientUnits=m*s*N/rad  TorqueActuationMode=NoTorque  MotionActuationMode=ComputedMotion  SensePosition=off  SenseVelocity=off  SenseAcceleration=off  SenseTorqueForce=off  SenseLowerLimitTorqueForce=off  SenseUpperLimitTorqueForce=off  LowerLimitSpecify=off  LowerLimitBound=-90  LowerLimitBoundUnits=deg  LowerLimitStiffness=1e4  LowerLimitStiffnessUnits=N*m/deg  LowerLimitDamping=10  LowerLimitDampingUnits=N*m/(deg/s)  LowerLimitTransitionRegionWidth=0.1  LowerLimitTransitionRegionWidthUnits=deg  UpperLimitSpecify=off  UpperLimitBound=90  UpperLimitBoundUnits=deg  UpperLimitStiffness=1e4  UpperLimitStiffnessUnits=N*m/deg  UpperLimitDamping=10  UpperLimitDampingUnits=N*m/(deg/s)  UpperLimitTransitionRegionWidth=0.1  UpperLimitTransitionRegionWidthUnits=deg  PositionTargetSpecify=on  PositionTargetPriority=Low  PositionTargetValue=-88.697456915883478  PositionTargetValueUnits=deg  VelocityTargetSpecify=off  VelocityTargetPriority=High  VelocityTargetValue=0  VelocityTargetValueUnits=deg/s
  Revolute9 : sm_lib/Joints/Revolute Joint  JointMode=Normal  SenseConstraintForce=off  SenseConstraintForceX=off  SenseConstraintForceY=off  SenseConstraintForceZ=off  SenseConstraintTorque=off  SenseConstraintTorqueX=off  SenseConstraintTorqueY=off  SenseConstraintTorqueZ=off  SenseTotalForce=off  SenseTotalForceX=off  SenseTotalForceY=off  SenseTotalForceZ=off  SenseTotalTorque=off  SenseTotalTorqueX=off  SenseTotalTorqueY=off  SenseTotalTorqueZ=off  CompositeWrenchDir=FollowerOnBase  CompositeWrenchFrame=BaseFrame  EquilibriumPosition=0  EquilibriumPositionUnits=rad  SpringStiffness=0  SpringStiffnessUnits=m*N/rad  DampingCoefficient=0  DampingCoefficientUnits=m*s*N/rad  TorqueActuationMode=NoTorque  MotionActuationMode=ComputedMotion  SensePosition=off  SenseVelocity=off  SenseAcceleration=off  SenseTorqueForce=off  SenseLowerLimitTorqueForce=off  SenseUpperLimitTorqueForce=off  LowerLimitSpecify=off  LowerLimitBound=-90  LowerLimitBoundUnits=deg  LowerLimitStiffness=1e4  LowerLimitStiffnessUnits=N*m/deg  LowerLimitDamping=10  LowerLimitDampingUnits=N*m/(deg/s)  LowerLimitTransitionRegionWidth=0.1  LowerLimitTransitionRegionWidthUnits=deg  UpperLimitSpecify=off  UpperLimitBound=90  UpperLimitBoundUnits=deg  UpperLimitStiffness=1e4  UpperLimitStiffnessUnits=N*m/deg  UpperLimitDamping=10  UpperLimitDampingUnits=N*m/(deg/s)  UpperLimitTransitionRegionWidth=0.1  UpperLimitTransitionRegionWidthUnits=deg  PositionTargetSpecify=on  PositionTargetPriority=Low  PositionTargetValue=91.30254308411601  PositionTargetValueUnits=deg  VelocityTargetSpecify=off  VelocityTargetPriority=High  VelocityTargetValue=0  VelocityTargetValueUnits=deg/s
  S1 : PMIOPort  Side=Right
  E1 : PMIOPort  Port=2  Side=Left
  Ref : PMIOPort  Port=3  Side=Left
  Ref1 : PMIOPort  Port=4  Side=Right
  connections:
  Interface1/RConn1 -- Revolute14/LConn2
  Interface1/LConn2 -- Ref/RConn1
  Interface1/RConn2 -- Revolute14/RConn2
  Interface1/LConn1 -- E1/RConn1
  BIELLE_5_RIGID/LConn1 -- Revolute8/LConn1
  BIELLE_6_RIGID/LConn1 -- Revolute10/LConn1
  JOINT_5_RIGID/LConn2 -- Revolute9/RConn1
  JOINT_3_RIGID/RConn1 -- Revolute10/RConn1
  JOINT_5_RIGID/LConn1 -- Revolute11/RConn1
  Ref1/RConn1 -- Revolute14/LConn1
  BRAS_3_RIGID/RConn1 -- Revolute17/LConn1
  BIELLE_5_RIGID/RConn1 -- Revolute9/LConn1
  JOINT_5_RIGID/RConn1 -- Revolute20/RConn1
  BIELLE_6_RIGID/RConn1 -- Revolute11/LConn1
  BRAS_3_RIGID/LConn1 -- Revolute14/RConn1
  S1/RConn1 -- Revolute20/LConn1
  JOINT_3_RIGID/RConn2 -- Revolute8/RConn1
  JOINT_3_RIGID/LConn1 -- Revolute17/RConn1

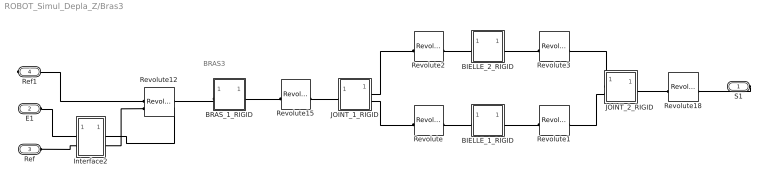
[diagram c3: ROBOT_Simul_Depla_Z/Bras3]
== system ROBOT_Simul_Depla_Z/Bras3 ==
  note: BRAS3
  BIELLE_1_RIGID : Subsystem
  BIELLE_2_RIGID : Subsystem
  BRAS_1_RIGID : Subsystem
  Interface2 : Subsystem
  JOINT_1_RIGID : Subsystem
  JOINT_2_RIGID : Subsystem
  Revolute : sm_lib/Joints/Revolute Joint  JointMode=Normal  SenseConstraintForce=off  SenseConstraintForceX=off  SenseConstraintForceY=off  SenseConstraintForceZ=off  SenseConstraintTorque=off  SenseConstraintTorqueX=off  SenseConstraintTorqueY=off  SenseConstraintTorqueZ=off  SenseTotalForce=off  SenseTotalForceX=off  SenseTotalForceY=off  SenseTotalForceZ=off  SenseTotalTorque=off  SenseTotalTorqueX=off  SenseTotalTorqueY=off  SenseTotalTorqueZ=off  CompositeWrenchDir=FollowerOnBase  CompositeWrenchFrame=BaseFrame  EquilibriumPosition=0  EquilibriumPositionUnits=rad  SpringStiffness=0  SpringStiffnessUnits=m*N/rad  DampingCoefficient=0  DampingCoefficientUnits=m*s*N/rad  TorqueActuationMode=NoTorque  MotionActuationMode=ComputedMotion  SensePosition=off  SenseVelocity=off  SenseAcceleration=off  SenseTorqueForce=off  SenseLowerLimitTorqueForce=off  SenseUpperLimitTorqueForce=off  LowerLimitSpecify=off  LowerLimitBound=-90  LowerLimitBoundUnits=deg  LowerLimitStiffness=1e4  LowerLimitStiffnessUnits=N*m/deg  LowerLimitDamping=10  LowerLimitDampingUnits=N*m/(deg/s)  LowerLimitTransitionRegionWidth=0.1  LowerLimitTransitionRegionWidthUnits=deg  UpperLimitSpecify=off  UpperLimitBound=90  UpperLimitBoundUnits=deg  UpperLimitStiffness=1e4  UpperLimitStiffnessUnits=N*m/deg  UpperLimitDamping=10  UpperLimitDampingUnits=N*m/(deg/s)  UpperLimitTransitionRegionWidth=0.1  UpperLimitTransitionRegionWidthUnits=deg  PositionTargetSpecify=on  PositionTargetPriority=Low  PositionTargetValue=91.302543084116763  PositionTargetValueUnits=deg  VelocityTargetSpecify=off  VelocityTargetPriority=High  VelocityTargetValue=0  VelocityTargetValueUnits=deg/s
  Revolute1 : sm_lib/Joints/Revolute Joint  JointMode=Normal  SenseConstraintForce=off  SenseConstraintForceX=off  SenseConstraintForceY=off  SenseConstraintForceZ=off  SenseConstraintTorque=off  SenseConstraintTorqueX=off  SenseConstraintTorqueY=off  SenseConstraintTorqueZ=off  SenseTotalForce=off  SenseTotalForceX=off  SenseTotalForceY=off  SenseTotalForceZ=off  SenseTotalTorque=off  SenseTotalTorqueX=off  SenseTotalTorqueY=off  SenseTotalTorqueZ=off  CompositeWrenchDir=FollowerOnBase  CompositeWrenchFrame=BaseFrame  EquilibriumPosition=0  EquilibriumPositionUnits=rad  SpringStiffness=0  SpringStiffnessUnits=m*N/rad  DampingCoefficient=0  DampingCoefficientUnits=m*s*N/rad  TorqueActuationMode=NoTorque  MotionActuationMode=ComputedMotion  SensePosition=off  SenseVelocity=off  SenseAcceleration=off  SenseTorqueForce=off  SenseLowerLimitTorqueForce=off  SenseUpperLimitTorqueForce=off  LowerLimitSpecify=off  LowerLimitBound=-90  LowerLimitBoundUnits=deg  LowerLimitStiffness=1e4  LowerLimitStiffnessUnits=N*m/deg  LowerLimitDamping=10  LowerLimitDampingUnits=N*m/(deg/s)  LowerLimitTransitionRegionWidth=0.1  LowerLimitTransitionRegionWidthUnits=deg  UpperLimitSpecify=off  UpperLimitBound=90  UpperLimitBoundUnits=deg  UpperLimitStiffness=1e4  UpperLimitStiffnessUnits=N*m/deg  UpperLimitDamping=10  UpperLimitDampingUnits=N*m/(deg/s)  UpperLimitTransitionRegionWidth=0.1  UpperLimitTransitionRegionWidthUnits=deg  PositionTargetSpecify=on  PositionTargetPriority=Low  PositionTargetValue=91.302543084117588  PositionTargetValueUnits=deg  VelocityTargetSpecify=off  VelocityTargetPriority=High  VelocityTargetValue=0  VelocityTargetValueUnits=deg/s
  Revolute12 : sm_lib/Joints/Revolute Joint  JointMode=Normal  SenseConstraintForce=off  SenseConstraintForceX=off  SenseConstraintForceY=off  SenseConstraintForceZ=off  SenseConstraintTorque=off  SenseConstraintTorqueX=off  SenseConstraintTorqueY=off  SenseConstraintTorqueZ=off  SenseTotalForce=off  SenseTotalForceX=off  SenseTotalForceY=off  SenseTotalForceZ=off  SenseTotalTorque=off  SenseTotalTorqueX=off  SenseTotalTorqueY=off  SenseTotalTorqueZ=off  CompositeWrenchDir=FollowerOnBase  CompositeWrenchFrame=BaseFrame  EquilibriumPosition=0  EquilibriumPositionUnits=rad  SpringStiffness=0  SpringStiffnessUnits=m*N/rad  DampingCoefficient=0  DampingCoefficientUnits=m*s*N/rad  TorqueActuationMode=InputTorque  MotionActuationMode=ComputedMotion  SensePosition=off  SenseVelocity=on  SenseAcceleration=off  SenseTorqueForce=off  SenseLowerLimitTorqueForce=off  SenseUpperLimitTorqueForce=off  LowerLimitSpecify=off  LowerLimitBound=-90  LowerLimitBoundUnits=deg  LowerLimitStiffness=1e4  LowerLimitStiffnessUnits=N*m/deg  LowerLimitDamping=10  LowerLimitDampingUnits=N*m/(deg/s)  LowerLimitTransitionRegionWidth=0.1  LowerLimitTransitionRegionWidthUnits=deg  UpperLimitSpecify=off  UpperLimitBound=90  UpperLimitBoundUnits=deg  UpperLimitStiffness=1e4  UpperLimitStiffnessUnits=N*m/deg  UpperLimitDamping=10  UpperLimitDampingUnits=N*m/(deg/s)  UpperLimitTransitionRegionWidth=0.1  UpperLimitTransitionRegionWidthUnits=deg  PositionTargetSpecify=on  PositionTargetPriority=Low  PositionTargetValue=-101.88737871174806  PositionTargetValueUnits=deg  VelocityTargetSpecify=off  VelocityTargetPriority=High  VelocityTargetValue=0  VelocityTargetValueUnits=deg/s
  Revolute15 : sm_lib/Joints/Revolute Joint  JointMode=Normal  SenseConstraintForce=off  SenseConstraintForceX=off  SenseConstraintForceY=off  SenseConstraintForceZ=off  SenseConstraintTorque=off  SenseConstraintTorqueX=off  SenseConstraintTorqueY=off  SenseConstraintTorqueZ=off  SenseTotalForce=off  SenseTotalForceX=off  SenseTotalForceY=off  SenseTotalForceZ=off  SenseTotalTorque=off  SenseTotalTorqueX=off  SenseTotalTorqueY=off  SenseTotalTorqueZ=off  CompositeWrenchDir=FollowerOnBase  CompositeWrenchFrame=BaseFrame  EquilibriumPosition=0  EquilibriumPositionUnits=rad  SpringStiffness=0  SpringStiffnessUnits=m*N/rad  DampingCoefficient=0  DampingCoefficientUnits=m*s*N/rad  TorqueActuationMode=NoTorque  MotionActuationMode=ComputedMotion  SensePosition=off  SenseVelocity=off  SenseAcceleration=off  SenseTorqueForce=off  SenseLowerLimitTorqueForce=off  SenseUpperLimitTorqueForce=off  LowerLimitSpecify=off  LowerLimitBound=-90  LowerLimitBoundUnits=deg  LowerLimitStiffness=1e4  LowerLimitStiffnessUnits=N*m/deg  LowerLimitDamping=10  LowerLimitDampingUnits=N*m/(deg/s)  LowerLimitTransitionRegionWidth=0.1  LowerLimitTransitionRegionWidthUnits=deg  UpperLimitSpecify=off  UpperLimitBound=90  UpperLimitBoundUnits=deg  UpperLimitStiffness=1e4  UpperLimitStiffnessUnits=N*m/deg  UpperLimitDamping=10  UpperLimitDampingUnits=N*m/(deg/s)  UpperLimitTransitionRegionWidth=0.1  UpperLimitTransitionRegionWidthUnits=deg  PositionTargetSpecify=on  PositionTargetPriority=Low  PositionTargetValue=-52.858992130052194  PositionTargetValueUnits=deg  VelocityTargetSpecify=off  VelocityTargetPriority=High  VelocityTargetValue=0  VelocityTargetValueUnits=deg/s
  Revolute18 : sm_lib/Joints/Revolute Joint  JointMode=Normal  SenseConstraintForce=off  SenseConstraintForceX=off  SenseConstraintForceY=off  SenseConstraintForceZ=off  SenseConstraintTorque=off  SenseConstraintTorqueX=off  SenseConstraintTorqueY=off  SenseConstraintTorqueZ=off  SenseTotalForce=off  SenseTotalForceX=off  SenseTotalForceY=off  SenseTotalForceZ=off  SenseTotalTorque=off  SenseTotalTorqueX=off  SenseTotalTorqueY=off  SenseTotalTorqueZ=off  CompositeWrenchDir=FollowerOnBase  CompositeWrenchFrame=BaseFrame  EquilibriumPosition=0  EquilibriumPositionUnits=rad  SpringStiffness=0  SpringStiffnessUnits=m*N/rad  DampingCoefficient=0  DampingCoefficientUnits=m*s*N/rad  TorqueActuationMode=NoTorque  MotionActuationMode=ComputedMotion  SensePosition=off  SenseVelocity=off  SenseAcceleration=off  SenseTorqueForce=off  SenseLowerLimitTorqueForce=off  SenseUpperLimitTorqueForce=off  LowerLimitSpecify=off  LowerLimitBound=-90  LowerLimitBoundUnits=deg  LowerLimitStiffness=1e4  LowerLimitStiffnessUnits=N*m/deg  LowerLimitDamping=10  LowerLimitDampingUnits=N*m/(deg/s)  LowerLimitTransitionRegionWidth=0.1  LowerLimitTransitionRegionWidthUnits=deg  UpperLimitSpecify=off  UpperLimitBound=90  UpperLimitBoundUnits=deg  UpperLimitStiffness=1e4  UpperLimitStiffnessUnits=N*m/deg  UpperLimitDamping=10  UpperLimitDampingUnits=N*m/(deg/s)  UpperLimitTransitionRegionWidth=0.1  UpperLimitTransitionRegionWidthUnits=deg  PositionTargetSpecify=on  PositionTargetPriority=Low  PositionTargetValue=-139.02838658169591  PositionTargetValueUnits=deg  VelocityTargetSpecify=off  VelocityTargetPriority=High  VelocityTargetValue=0  VelocityTargetValueUnits=deg/s
  Revolute2 : sm_lib/Joints/Revolute Joint  JointMode=Normal  SenseConstraintForce=off  SenseConstraintForceX=off  SenseConstraintForceY=off  SenseConstraintForceZ=off  SenseConstraintTorque=off  SenseConstraintTorqueX=off  SenseConstraintTorqueY=off  SenseConstraintTorqueZ=off  SenseTotalForce=off  SenseTotalForceX=off  SenseTotalForceY=off  SenseTotalForceZ=off  SenseTotalTorque=off  SenseTotalTorqueX=off  SenseTotalTorqueY=off  SenseTotalTorqueZ=off  CompositeWrenchDir=FollowerOnBase  CompositeWrenchFrame=BaseFrame  EquilibriumPosition=0  EquilibriumPositionUnits=rad  SpringStiffness=0  SpringStiffnessUnits=m*N/rad  DampingCoefficient=0  DampingCoefficientUnits=m*s*N/rad  TorqueActuationMode=NoTorque  MotionActuationMode=ComputedMotion  SensePosition=off  SenseVelocity=off  SenseAcceleration=off  SenseTorqueForce=off  SenseLowerLimitTorqueForce=off  SenseUpperLimitTorqueForce=off  LowerLimitSpecify=off  LowerLimitBound=-90  LowerLimitBoundUnits=deg  LowerLimitStiffness=1e4  LowerLimitStiffnessUnits=N*m/deg  LowerLimitDamping=10  LowerLimitDampingUnits=N*m/(deg/s)  LowerLimitTransitionRegionWidth=0.1  LowerLimitTransitionRegionWidthUnits=deg  UpperLimitSpecify=off  UpperLimitBound=90  UpperLimitBoundUnits=deg  UpperLimitStiffness=1e4  UpperLimitStiffnessUnits=N*m/deg  UpperLimitDamping=10  UpperLimitDampingUnits=N*m/(deg/s)  UpperLimitTransitionRegionWidth=0.1  UpperLimitTransitionRegionWidthUnits=deg  PositionTargetSpecify=on  PositionTargetPriority=Low  PositionTargetValue=-88.697456915883265  PositionTargetValueUnits=deg  VelocityTargetSpecify=off  VelocityTargetPriority=High  VelocityTargetValue=0  VelocityTargetValueUnits=deg/s
  Revolute3 : sm_lib/Joints/Revolute Joint  JointMode=Normal  SenseConstraintForce=off  SenseConstraintForceX=off  SenseConstraintForceY=off  SenseConstraintForceZ=off  SenseConstraintTorque=off  SenseConstraintTorqueX=off  SenseConstraintTorqueY=off  SenseConstraintTorqueZ=off  SenseTotalForce=off  SenseTotalForceX=off  SenseTotalForceY=off  SenseTotalForceZ=off  SenseTotalTorque=off  SenseTotalTorqueX=off  SenseTotalTorqueY=off  SenseTotalTorqueZ=off  CompositeWrenchDir=FollowerOnBase  CompositeWrenchFrame=BaseFrame  EquilibriumPosition=0  EquilibriumPositionUnits=rad  SpringStiffness=0  SpringStiffnessUnits=m*N/rad  DampingCoefficient=0  DampingCoefficientUnits=m*s*N/rad  TorqueActuationMode=NoTorque  MotionActuationMode=ComputedMotion  SensePosition=off  SenseVelocity=off  SenseAcceleration=off  SenseTorqueForce=off  SenseLowerLimitTorqueForce=off  SenseUpperLimitTorqueForce=off  LowerLimitSpecify=off  LowerLimitBound=-90  LowerLimitBoundUnits=deg  LowerLimitStiffness=1e4  LowerLimitStiffnessUnits=N*m/deg  LowerLimitDamping=10  LowerLimitDampingUnits=N*m/(deg/s)  LowerLimitTransitionRegionWidth=0.1  LowerLimitTransitionRegionWidthUnits=deg  UpperLimitSpecify=off  UpperLimitBound=90  UpperLimitBoundUnits=deg  UpperLimitStiffness=1e4  UpperLimitStiffnessUnits=N*m/deg  UpperLimitDamping=10  UpperLimitDampingUnits=N*m/(deg/s)  UpperLimitTransitionRegionWidth=0.1  UpperLimitTransitionRegionWidthUnits=deg  PositionTargetSpecify=off  PositionTargetPriority=High  PositionTargetValue=0  PositionTargetValueUnits=deg  VelocityTargetSpecify=off  VelocityTargetPriority=High  VelocityTargetValue=0  VelocityTargetValueUnits=deg/s
  S1 : PMIOPort  Side=Right
  E1 : PMIOPort  Port=2  Side=Left
  Ref : PMIOPort  Port=3  Side=Left
  Ref1 : PMIOPort  Port=4  Side=Right
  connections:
  JOINT_1_RIGID/RConn2 -- Revolute/LConn1
  BRAS_1_RIGID/RConn1 -- Revolute15/LConn1
  Ref1/RConn1 -- Revolute12/RConn1
  S1/RConn1 -- Revolute18/RConn1
  JOINT_1_RIGID/LConn1 -- Revolute15/RConn1
  BIELLE_1_RIGID/LConn1 -- Revolute/RConn1
  BIELLE_1_RIGID/RConn1 -- Revolute1/LConn1
  BRAS_1_RIGID/LConn1 -- Revolute12/LConn1
  JOINT_2_RIGID/RConn1 -- Revolute18/LConn1
  JOINT_2_RIGID/LConn2 -- Revolute1/RConn1
  BIELLE_2_RIGID/LConn1 -- Revolute2/RConn1
  JOINT_1_RIGID/RConn1 -- Revolute2/LConn1
  JOINT_2_RIGID/LConn1 -- Revolute3/RConn1
  BIELLE_2_RIGID/RConn1 -- Revolute3/LConn1
  Interface2/LConn2 -- Ref/RConn1
  Interface2/RConn2 -- Revolute12/RConn2
  Interface2/RConn1 -- Revolute12/LConn2
  E1/RConn1 -- Interface2/LConn1
